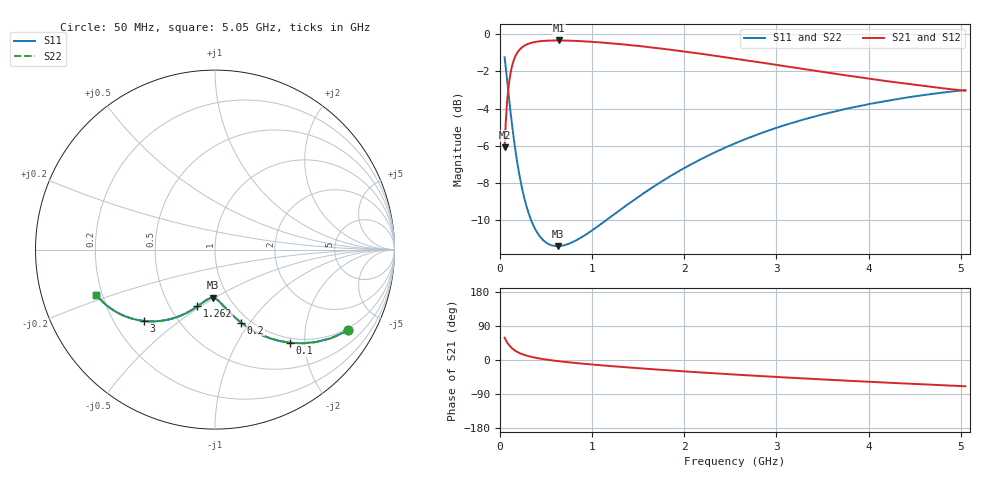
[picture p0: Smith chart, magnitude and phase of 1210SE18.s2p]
! AVX Thin Film Operation		Date: August 2001
! Description: Accu-P® Series, Thin Film, SMD, RF Capacitor
! Part Number: 12101J180FBT
! 50 MHz  -  5.05 GHz
! Serial Measurements
# mhz S db R 50
!	S11		S21		S12		S22
!	dB	Phase	dB	Phase	dB	Phase	dB	Phase
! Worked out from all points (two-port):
!   401 points, 50 MHz to 5.05 GHz, reference 50 ohm
!   highest |S21| = -0.33 dB at 637.5 MHz (marker M1); lowest = -6.1 dB at 50 MHz (marker M2)
!   |S21| within 3 dB of the highest: 82.95 MHz to end of sweep
!   lowest |S11| = -11.4 dB at 625 MHz (marker M3), VSWR 1.74, Z = 42.2 - j24.5 ohm
!   |S11| at or under -10 dB: 337.3 MHz to 1.155 GHz (817.9 MHz wide, 110 % of centre)
!   |S22| runs from -11.4 to -1.2 dB; largest |S21 - S12| = 0
!   S11 on the Smith chart (normalised r, x): 50 MHz: 0.92, -3.35; 100 MHz: 0.91, -1.70; 200 MHz: 0.91, -0.91; 1.262 GHz: 0.68, -0.48; 3 GHz: 0.33, -0.38; 5.05 GHz: 0.18, -0.18
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50  -1.23 -31.2  -6.08 58.8  -6.08 58.8  -1.23 -31.2
75  -2.37 -42.6  -3.77 47.4  -3.77 47.4  -2.37 -42.6
100  -3.54 -51.2  -2.54 38.8  -2.54 38.8  -3.54 -51.2
125  -4.64 -57.8  -1.83 32.2  -1.83 32.2  -4.64 -57.8
150  -5.63 -62.9  -1.39 27.1  -1.39 27.1  -5.63 -62.9
175  -6.51 -67.0  -1.10 23.0  -1.10 23.0  -6.51 -67.0
200  -7.29 -70.3  -0.90 19.7  -0.90 19.7  -7.29 -70.3
237.5  -8.26 -74.3  -0.70 15.7  -0.70 15.7  -8.26 -74.3
275  -9.04 -77.4  -0.58 12.5  -0.58 12.5  -9.04 -77.4
375  -10.42 -83.5  -0.41 6.4  -0.41 6.4  -10.42 -83.5
487.5  -11.17 -88.3  -0.35 1.6  -0.35 1.6  -11.17 -88.3
625  -11.41 -92.8  -0.33 -2.8  -0.33 -2.8  -11.41 -92.8
637.5  -11.40 -93.1  -0.33 -3.2  -0.33 -3.2  -11.40 -93.1
887.5  -10.92 -99.4  -0.37 -9.5  -0.37 -9.5  -10.92 -99.4
1262.5  -9.61 -107.2  -0.51 -17.2  -0.51 -17.2  -9.61 -107.2
1725  -8.01 -115.5  -0.75 -25.5  -0.75 -25.5  -8.01 -115.5
2125  -6.86 -122.0  -1.01 -32.0  -1.01 -32.0  -6.86 -122.0
2550  -5.87 -128.4  -1.31 -38.4  -1.31 -38.4  -5.87 -128.4
3000  -5.03 -134.7  -1.64 -44.8  -1.64 -44.8  -5.03 -134.7
3387.5  -4.46 -139.9  -1.94 -49.9  -1.94 -49.9  -4.46 -139.9
4225  -3.56 -150.0  -2.54 -60.1  -2.54 -60.1  -3.56 -150.0
5050  -3.00 -159.2  -3.04 -69.3  -3.04 -69.3  -3.00 -159.2
